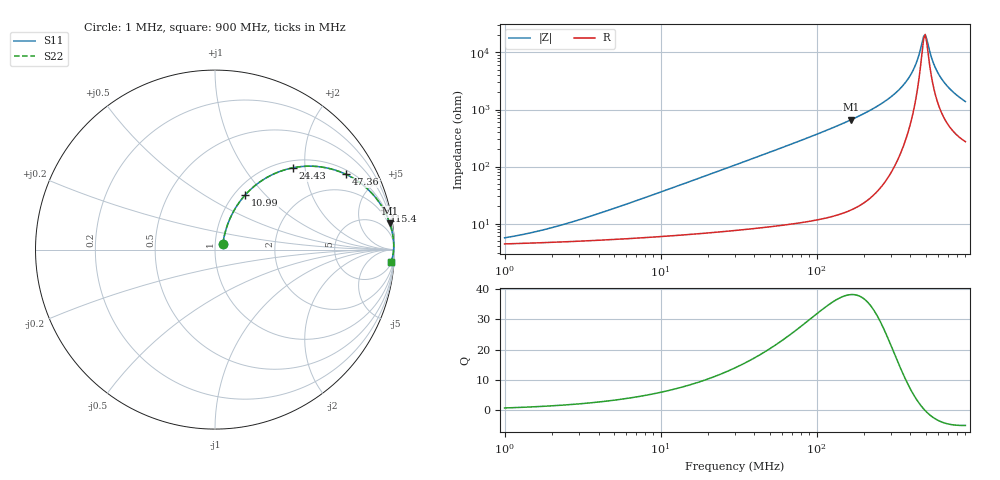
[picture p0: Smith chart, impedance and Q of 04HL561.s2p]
! Coilcraft 0402HL-561 Chip Inductor
! 20 July 2012
# MHz S MA R 50
!Freq  MagS11  AngS11  MagS21  AngS21  MagS12  AngS12  MagS22  AngS22
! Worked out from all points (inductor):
!   299 points, 1 MHz to 900 MHz, reference 50 ohm
!   read as one part in series: L = 560 nH near 4.409 MHz
!   highest Q = 38.1 at 166.2 MHz (marker M1), where L = 631 nH
!   self-resonance near 485.9 MHz
!   S11 on the Smith chart (normalised r, x): 1 MHz: 1.09, +0.07; 10.99 MHz: 1.12, +0.77; 24.43 MHz: 1.14, +1.72; 47.36 MHz: 1.17, +3.36; 115.4 MHz: 1.25, +8.58; 900 MHz: 6, -27
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1  0.05393 36.7  0.9573 -1.9  0.9573 -1.9  0.05393 36.7
1.72952  0.07291 49.5  0.9542 -3.3  0.9542 -3.3  0.07291 49.5
3.130965  0.1144 59.9  0.9477 -6.0  0.9477 -6.0  0.1144 59.9
9.802945  0.3143 62.3  0.8979 -18.0  0.8979 -18.0  0.3143 62.3
10.98814  0.3469 61.1  0.8861 -20.0  0.8861 -20.0  0.3469 61.1
16.19776  0.4752 55.3  0.8275 -28.2  0.8275 -28.2  0.4752 55.3
24.42863  0.6287 46.4  0.7272 -38.8  0.7272 -38.8  0.6287 46.4
30.69268  0.7115 40.8  0.6547 -45.2  0.6547 -45.2  0.7115 40.8
47.35791  0.8411 29.9  0.4995 -57.1  0.4995 -57.1  0.8411 29.9
93.92896  0.9517 16.1  0.2774 -72.0  0.2774 -72.0  0.9517 16.1
115.3511  0.9677 13.0  0.2254 -75.3  0.2254 -75.3  0.9677 13.0
166.2029  0.9849 8.6  0.1494 -79.9  0.1494 -79.9  0.9849 8.6
294.0883  0.9953 3.6  0.06226 -83.9  0.06226 -83.9  0.9953 3.6
353.0094  0.9961 2.3  0.03954 -83.3  0.03954 -83.3  0.9961 2.3
404.8254  0.9962 1.3  0.02349 -79.9  0.02349 -79.9  0.9962 1.3
443.529  0.9959 0.7  0.01332 -71.6  0.01332 -71.6  0.9959 0.7
485.9328  0.9954 0.1  0.005166 -26.2  0.005166 -26.2  0.9954 0.1
497.1527  0.9952 -0.0  0.004812 3.6  0.004812 3.6  0.9952 -0.0
557.2597  0.9941 -0.8  0.01446 65.5  0.01446 65.5  0.9941 -0.8
610.5369  0.9929 -1.4  0.02461 72.5  0.02461 72.5  0.9929 -1.4
716.3196  0.9899 -2.4  0.04315 75.3  0.04315 75.3  0.9899 -2.4
900  0.9834 -4.0  0.0713 74.6  0.0713 74.6  0.9834 -4.0
